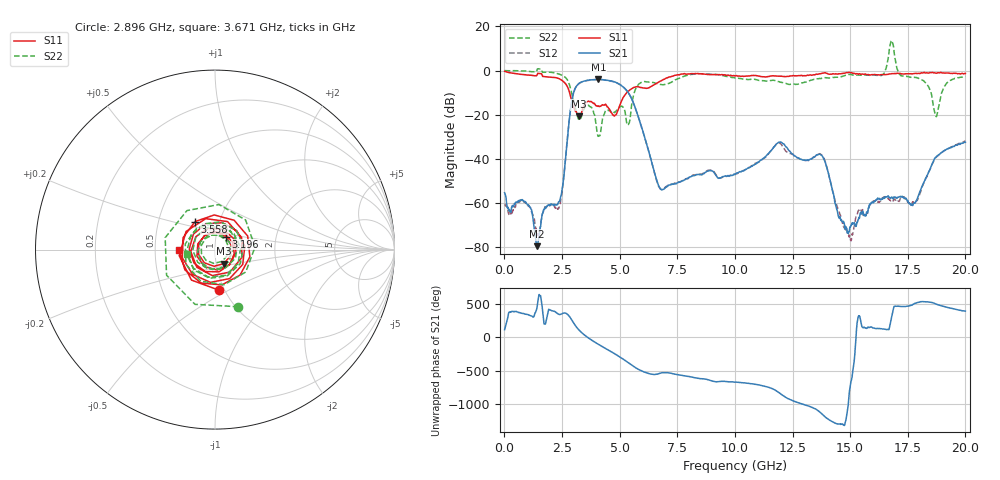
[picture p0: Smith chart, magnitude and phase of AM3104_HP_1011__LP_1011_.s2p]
!Created with skrf (http://scikit-rf.org).
# Hz S RI R 50.0
!freq ReS11 ImS11 ReS21 ImS21 ReS12 ImS12 ReS22 ImS22
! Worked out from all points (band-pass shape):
!   1601 points, 10 MHz to 20 GHz, reference 50 ohm
!   highest |S21| = -4.04 dB at 4.083 GHz (marker M1); lowest = -79.7 dB at 1.422 GHz (marker M2)
!   |S21| within 3 dB of the highest: 3.13 GHz to 5.107 GHz (1.977 GHz wide, 48 % of centre)
!   lowest |S11| = -20.7 dB at 3.233 GHz (marker M3), VSWR 1.20, Z = 54.4 - j8.61 ohm
!   |S11| at or under -10 dB: 2.828 GHz to 5.313 GHz (2.485 GHz wide, 61.1 % of centre)
!   |S22| runs from -29.9 to 13.6 dB; largest |S21 - S12| = 0.052
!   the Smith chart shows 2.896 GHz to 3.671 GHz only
!   S11 on the Smith chart (normalised r, x): 2.896 GHz: 0.94, -0.45; 3.196 GHz: 1.12, +0.16; 3.558 GHz: 0.77, +0.25; 3.671 GHz: 0.67, -0.00
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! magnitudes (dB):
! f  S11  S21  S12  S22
! 10 MHz  -0.3  -55.4  -60.5  -0.1
! 1.084 GHz  -2.1  -61.5  -61.9  -0.4
! 1.422 GHz  -1.9  -79.7  -73.9  0.4
! 2.409 GHz  -3.9  -58.7  -60.6  -1.8
! 2.896 GHz  -12.9  -15.7  -15.8  -9.3
! 3.196 GHz  -20.5  -6.3  -6.3  -21.5
! 3.233 GHz  -20.7  -5.9  -6.0  -22.4
! 3.346 GHz  -19.2  -5.2  -5.3  -20.9
! 3.558 GHz  -14.3  -4.5  -4.6  -16.1
! 3.671 GHz  -14.0  -4.4  -4.5  -15.9
! 4.083 GHz  -16.0  -4.0  -4.1  -29.6
! 5.445 GHz  -8.8  -11.2  -11.2  -22.5
! 6.682 GHz  -5.3  -52.1  -52.3  -6.1
! 10.01 GHz  -2.5  -47.2  -47.1  -3.4
! 11.93 GHz  -2.5  -32.5  -32.8  -5.1
! 13.34 GHz  -2.1  -40.0  -39.9  -4.3
! 13.85 GHz  -1.1  -40.0  -39.6  -3.4
! 14.98 GHz  -0.9  -71.8  -74.8  -1.8
! 16.68 GHz  -1.6  -57.4  -58.4  7.2
! 17.78 GHz  -1.4  -60.1  -60.0  -3.1
! 18.73 GHz  -1.2  -39.3  -39.4  -20.8
! 20 GHz  -1.4  -32.5  -32.0  -2.7
